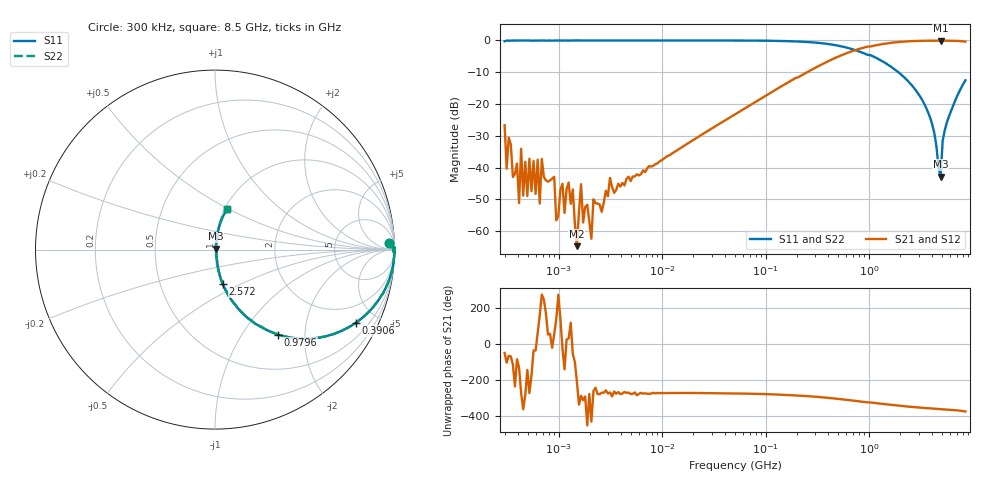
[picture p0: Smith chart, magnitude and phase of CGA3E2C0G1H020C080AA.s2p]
! S-parameter Generated by TDK Corporation
! Copyright(C) 2015 TDK Corporation.
! All Rights Reserved.
! TDK P/N: CGA3E2C0G1H020C080AA (Multilayer Ceramic Chip Capacitors)
! Property: C=2pF
! Size(LxWxT): 1.6x0.8x0.8mm, 0.063x0.031x0.031inches
! Model Type: s2p (Touchstone File Format Version 1.0)
! Frequency: DC=Yes Start=0.3MHz Stop=8500MHz 225points Log-sweep
! Note:
! Model Generated on Jun. 23, 2015
! Hash(MD5):
! Port Assignments:
!  1 ---| |--- 2
! Applicable Conditions:
!  Temperature = 25 degC
!  DC Bias Voltage = 0 V
!  Small Signal Operation
! Terms and conditions regarding TDK Simulation Models
! (1)This simulation model is being provided solely for informational purposes. Please refer to the specifications of the products in terms of detailed characteristics of such products.
! (2)In no event shall TDK Corporation of any of its subsidiaries be liable for any loss or damage arising, directly or indirectly,
!  From any information contained in this simulation model, including, but not limited to loss or damages arising from any inaccuracies, omissions or errors in connection with such information.
! (3)Any and all copyrights on this simulation model are owned by TDK Corporation.
!  Duplication or redistribution of this simulation model without prior written permission from TDK Corporation is prohibited.
! (4)This simulation model is subject to any modification or change without any prior notice.
! (5)Neither TDK Corporation nor any of its subsidiaries shall make any warranty, express or implied,
!  Including but not limited to the correctness, implied warranties of merchantability and fitness for a particular purpose with respect to this simulation models.
! (6)The use of this simulation model shall be deemed to have consented to the terms and conditions hereof.
# MHz S MA R 50
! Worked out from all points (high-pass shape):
!   224 points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, 300 kHz to 8.5 GHz, reference 50 ohm
!   highest |S21| = -0.04 dB at 4.896 GHz (marker M1); lowest = -64.7 dB at 1.499 MHz (marker M2)
!   |S21| within 3 dB of the highest: 733.1 MHz to end of sweep
!   lowest |S11| = -42.8 dB at 4.896 GHz (marker M3), VSWR 1.01, Z = 50.5 + j0.538 ohm
!   |S11| at or under -10 dB: 1.913 GHz to end of sweep
!   |S22| runs from -42.8 to 0.0 dB; largest |S21 - S12| = 6.7e-11
!   S11 on the Smith chart (normalised r, x): 300 kHz: 26, +33; 390.6 MHz: 1.02, -3.84; 979.6 MHz: 1.01, -1.47; 2.572 GHz: 1.01, -0.41; 8.5 GHz: 1.03, +0.49
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0.3  0.9713 2.1  0.04637 -50.7  0.04637 -50.7  0.9713 2.1
0.4138848  0.9982 0.1  0.002763 -131.3  0.002763 -131.3  0.9982 0.1
0.4333561  0.9996 -1.1  0.01977 88.2  0.01977 88.2  0.9996 -1.1
0.4537435  0.9964 -0.0  0.003617 -1.3  0.003617 -1.3  0.9964 -0.0
0.6259918  0.9937 -0.7  0.01331 61.8  0.01331 61.8  0.9937 -0.7
0.6554417  0.9975 -0.0  0.002721 156.9  0.002721 156.9  0.9975 -0.0
0.6862772  0.9995 0.8  0.01366 -88.0  0.01366 -88.0  0.9995 0.8
0.9042579  0.9956 -0.3  0.007146 52.0  0.007146 52.0  0.9956 -0.3
0.9467989  0.9989 -0.1  0.001478 135.2  0.001478 135.2  0.9989 -0.1
1.36767  0.9975 0.2  0.004527 -56.3  0.004527 -56.3  0.9975 0.2
1.499382  0.9995 -0.0  0.0005794 149.8  0.0005794 149.8  0.9995 -0.0
1.643778  0.9984 -0.3  0.005472 72.9  0.005472 72.9  0.9984 -0.3
1.72111  0.9991 -0.0  0.001365 48.5  0.001365 48.5  0.9991 -0.0
9.430415  0.9995 -0.7  0.0125 87.3  0.0125 87.3  0.9995 -0.7
51.67171  0.9971 -4.0  0.07017 85.6  0.07017 85.6  0.9971 -4.0
283.1228  0.9338 -20.6  0.3518 69.0  0.3518 69.0  0.9338 -20.6
390.6008  0.8846 -27.4  0.4608 62.2  0.4608 62.2  0.8846 -27.4
979.5854  0.5901 -53.4  0.8023 36.2  0.8023 36.2  0.5901 -53.4
1551.304  0.4061 -65.4  0.9095 24.0  0.9095 24.0  0.4061 -65.4
2572.272  0.1982 -77.1  0.9752 11.4  0.9752 11.4  0.1982 -77.1
4895.91  0.007228 47.4  0.9951 -0.3  0.9951 -0.3  0.007228 47.4
8500  0.2363 73.1  0.9585 -13.6  0.9585 -13.6  0.2363 73.1
